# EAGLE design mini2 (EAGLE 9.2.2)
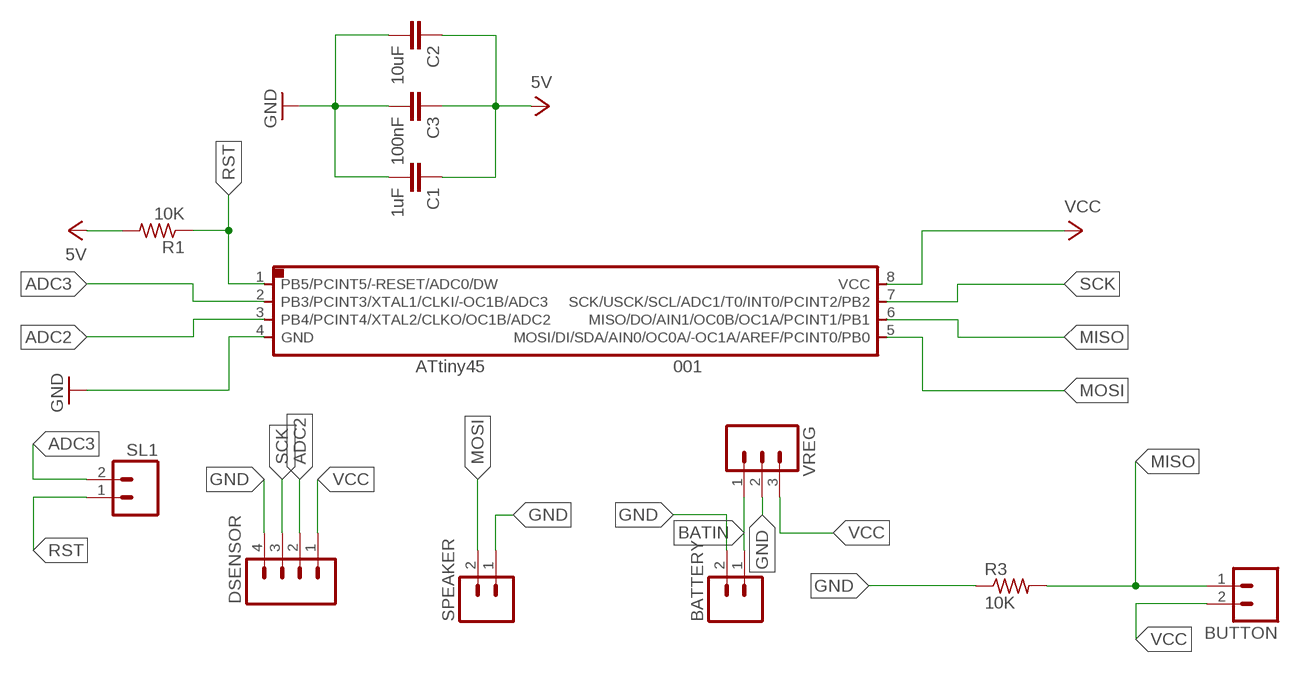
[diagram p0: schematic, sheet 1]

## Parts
001  ATTINY45SI  [SOIC8]
BATTERY  M02  [02P]
BUTTON  M02  [02P]
C1  1uF  CAP1206  [1206]
C2  10uF  CAP1206  [1206]
C3  100nF  CAP1206  [1206]
DSENSOR  M04  [04P]
R1  10K  RES-US1206FAB  [R1206FAB]
R3  10K  RES-US1206  [R1206]
SL1  M02  [02P]
SPEAKER  M02  [02P]
VREG  M03  [03P]

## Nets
ADC2: 001.3(PB4/PCINT4/XTAL2/CLKO/OC1B/ADC2) DSENSOR.2
ADC3: 001.2(PB3/PCINT3/XTAL1/CLKI/-OC1B/ADC3) SL1.2
BATIN: BATTERY.1 VREG.1
GND: 001.4(GND) BATTERY.2 C1.2 C2.2 C3.2 DSENSOR.4 R3.1 SPEAKER.1 VREG.2
MISO: 001.6(MISO/DO/AIN1/OC0B/OC1A/PCINT1/PB1) BUTTON.1 R3.2
MOSI: 001.5(MOSI/DI/SDA/AIN0/OC0A/-OC1A/AREF/PCINT0/PB0) SPEAKER.2
RST: 001.1(PB5/PCINT5/-RESET/ADC0/DW) R1.1 SL1.1
SCK: 001.7(SCK/USCK/SCL/ADC1/T0/INT0/PCINT2/PB2) DSENSOR.3
VCC: 001.8(VCC) BUTTON.2 C1.1 C2.1 C3.1 DSENSOR.1 R1.2 VREG.3 ; supply symbol labelled 5V

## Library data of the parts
001 = fab:ATTINY45
BATTERY BUTTON SL1 SPEAKER = con-amp-quick:M02: AMP QUICK CONNECTOR; OC_FARNELL: unknown; OC_NEWARK: unknown
C1-C3 = 01_SparkFun:CAP: Capacitor
DSENSOR = con-amp-quick:M04: AMP QUICK CONNECTOR; OC_FARNELL: unknown; OC_NEWARK: unknown
R1 R3 = fab:RES-US: Resistor (US Symbol)
VREG = con-amp-quick:M03: AMP QUICK CONNECTOR; OC_FARNELL: unknown; OC_NEWARK: unknown

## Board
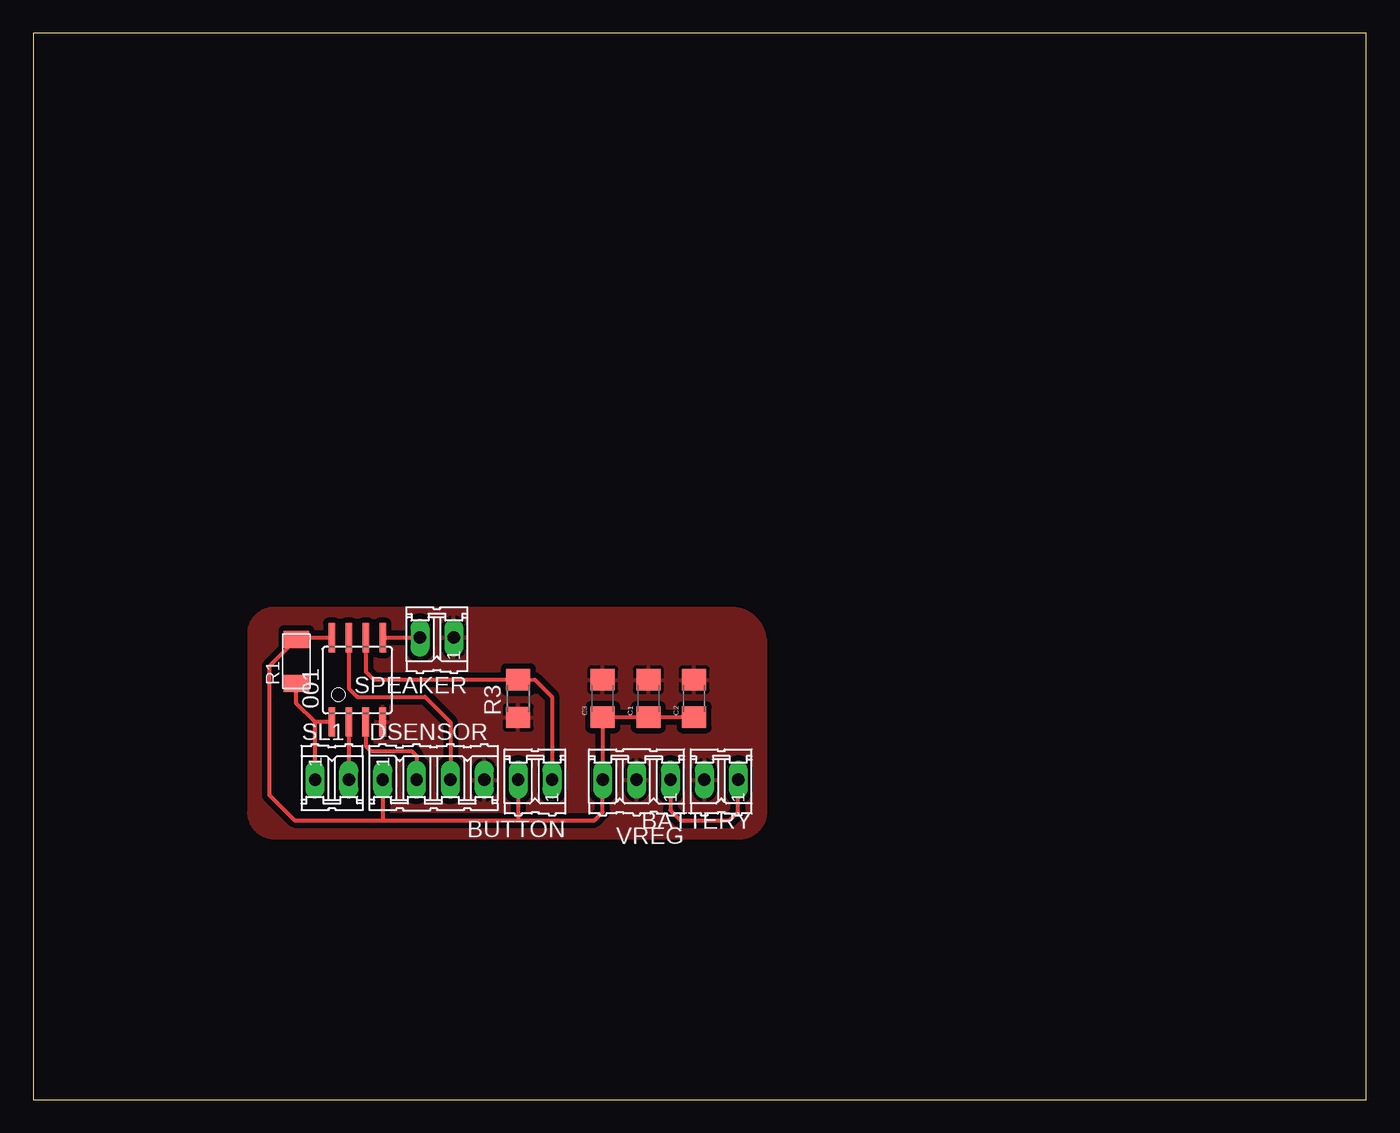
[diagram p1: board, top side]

Size 100 x 80 mm. Coordinates in mm from the lower left corner, seen from the top.
Outline: 100,80 0,80 0,0 100,0 100,80
Copper layers (1*16): Top 0.035mm / dielectric 1.5mm / Bottom 0.035mm
Design rules "default": minimum track width 10mil, minimum drill 24mil, track to track 8mil, track to pad 8mil, pad to pad 8mil, via to via 8mil, smd to smd 8mil, copper to edge 40mil, drill to drill 8mil, minimum pad ring 10mil, minimum via ring 8mil, stop-mask expansion 4mil, vias tented up to drill 0mil, thermal gap 10mil

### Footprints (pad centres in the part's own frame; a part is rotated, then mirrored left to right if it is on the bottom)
SOIC8 = smd 0.5 x 2.2: 1 -1.905,-3.154; 2 -0.645,-3.154; 3 0.625,-3.154; 4 1.895,-3.154; 5 1.905,3.154; 6 0.635,3.154; 7 -0.635,3.154; 8 -1.905,3.154
02P = drill 0.914 long: 1 -1.27,0; 2 1.27,0
1206 = smd 1.6 x 1.8: 1 -1.4,0; 2 1.4,0
04P = drill 0.914 long: 1 -3.81,0; 2 -1.27,0; 3 1.27,0; 4 3.81,0
R1206FAB = smd 1.27 x 1.905: 1 -1.651,0; 2 1.651,0
R1206 = smd 1.6 x 1.803: 1 -1.422,0; 2 1.422,0
03P = drill 0.914 long: 1 -2.54,0; 2 0,0; 3 2.54,0

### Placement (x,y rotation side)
001  24.31,31.49 0 top
BATTERY  51.61,23.99 180 top
BUTTON  37.64,23.99 180 top
C1  46.15,30.09 90 top
C2  49.58,30.09 90 top
C3  42.72,30.09 90 top
DSENSOR  30.02,23.99 0 top
R1  19.74,32.88 90 top
R3  36.37,30.09 90 top
SL1  22.4,23.99 0 top
SPEAKER  30.28,34.66 180 top
VREG  45.26,23.99 180 top

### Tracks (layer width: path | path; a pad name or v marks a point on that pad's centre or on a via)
ADC2
  Top 0.305: 001.3 24.93,26.54 25.32,26.15 28.37,26.15 28.75,25.77 DSENSOR.2
ADC3
  Top 0.305: 001.2 23.66,24 SL1.2
BATIN
  Top 0.305: VREG.1 47.8,21.71 48.57,20.94 52.25,20.94 52.88,21.58 BATTERY.1
GND
  Top 0.305: 26.21,28.34 001.4
  pour Top (isolate 0.406): 16.18,21.58 arc90 18.09,19.67 53.01,19.67 arc90 54.91,21.58 54.91,34.28 arc90 52.38,36.82 18.09,36.82 arc90 16.18,34.91
MISO
  Top 0.305: 001.6 24.94,32.12 25.58,31.49 36.22,31.49 R3.2 37.63,31.49 38.91,30.22 BUTTON.1
MOSI
  Top 0.305: 001.5 26.23,34.66 SPEAKER.2
RST
  Top 0.305: 001.1 21.13,28.33 | SL1.1 21.13,28.33 | 21.13,28.33 19.74,29.73 R1.1
SCK
  Top 0.305: 001.7 23.67,30.85 24.31,30.22 29.39,30.22 31.29,28.31 DSENSOR.3
VCC
  Top 0.254: 49.58,28.43 arc90 49.33,28.69
  Top 0.305: 001.8 19.83,34.64 R1.2 17.7,32.5 17.7,22.85 19.61,20.94 26.21,20.94 | C2.1 49.33,28.69 C1.1 C3.1 VREG.3 42.72,21.58 42.09,20.94 36.37,20.94 | 26.21,20.94 26.34,20.94 36.37,20.94 | DSENSOR.1 26.21,20.94 | BUTTON.2 36.37,20.94

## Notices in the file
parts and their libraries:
01_SparkFun: Licensing: CC v3.0 Share-Alike You are welcome to use this library for commercial purposes.
